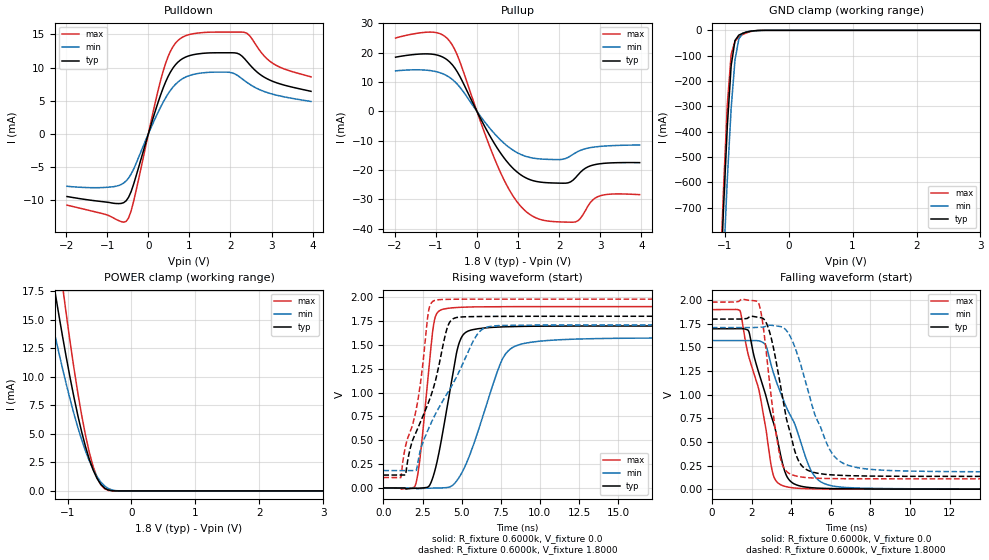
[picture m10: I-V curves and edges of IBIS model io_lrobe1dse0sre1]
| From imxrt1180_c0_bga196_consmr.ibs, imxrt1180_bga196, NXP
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[Model]  io_lrobe1dse0sre1
|   Model io_lrobe1dse0sre1
| This model was characterised for following simulation conditions:
| External (pad) voltage:
|   - Typ: 1.8V,   - Min: 1.71V,   - Max: 1.98V
| Library cells for typ/min/max conditions are connected as defined below:
|  PAD_IO - External Pad
|  ipp_do - Core Input
|  ipp_obe - Output Buffer Enable
|  ASRCN3V3[3] - NC
|  ASRCN3V3[4] - NC
|  ASRCP3V3[4] - NC
|  REFAPBIAS3V3 - gnde
|  REFBAMPL3V3 - vdd1v8
|  REFCAMPH3V3 - vdd1v8
|  REFDNBIAS3V3 - vdd1v8
|  REFH3V3 - REFH3V3
|  REFL3V3 - REFL3V3
|  gnde - gnde
|  ipp_dse - gnde
|  ipp_ina235_3v - NC
|  ipp_ina40_3v - NC
|  ipp_ina_mux - NC
|  ipp_ind - NC
|  ipp_ind_1p8v - NC
|  ipp_ind_3v - NC
|  ipp_sre - vdd
|  vdd - vdd
|  vdd1v8 - vdd1v8
|  vdda - vdde3v3
|  vdde3v3 - vdde3v3
| All other pins connected to ground
Model_type I/O
Polarity   Non-Inverting
Enable   Active-High
Vinl =   0.5400V
Vinh =   1.2600V
Vmeas =  0.9000V
Cref =   15.0000pF
Rref =   0.6000k
Vref =   0.0V
C_comp   3.9800pF   3.7960pF   4.1051pF
|C_comp_pullup   0.3206pF   0.4279pF   0.2788pF
|C_comp_pulldown   2.2503pF   2.3237pF   2.0515pF
[Model Spec]
| variable   typ   min   max
Vinh   1.2600V   NA   NA
Vinl   0.5400V   NA   NA
Vref   0.0V   0.0V   0.0V
Cref   15.0000pF   15.0000pF   15.0000pF
Rref   0.6000k   0.6000k   0.6000k
[Receiver Thresholds]
Vcross_high  =   0.0V
Vcross_low  =   0.0V
Vdiff_ac  =   0.0V
Vdiff_dc  =   0.0V
Tdiffslew_ac  =   0.0S
[Temperature Range]   25.0000   0.1250k   -40.0000
[Voltage Range]   1.8000V   1.7100V   1.9800V
[Pullup Reference]   1.8000V   1.7100V   1.9800V
[Pulldown Reference]   0.0V   0.0V   0.0V
[POWER Clamp Reference]   1.8000V   1.7100V   1.9800V
[GND Clamp Reference]   0.0V   0.0V   0.0V
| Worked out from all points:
|   slope of the pulldown table from 0 to 0.27 V, typ, clamps not added: 50.4 ohm
|   slope of the pullup table from 0 to 0.27 V, typ, clamps not added: 37.3 ohm
|   GND clamp passes 1 mA (typ) near -0.50 V on its own axis
|   POWER clamp passes 1 mA (typ) near -0.53 V on its own axis
|   rising waveform, R_fixture 0.6000k, V_fixture 0.0: 20-80 % time 1.09ns typ, 1.92ns min, 679ps max; typ from 0 V to 1.7 V
|   rising waveform, R_fixture 0.6000k, V_fixture 1.8000: 20-80 % time 1.97ns typ, 2.8ns min, 1.22ns max; typ from 0.135 V to 1.8 V
|   falling waveform, R_fixture 0.6000k, V_fixture 0.0: 20-80 % time 1.3ns typ, 1.7ns min, 1.16ns max; typ from 1.7 V to 0 V
|   falling waveform, R_fixture 0.6000k, V_fixture 1.8000: 20-80 % time 966ps typ, 1.43ns min, 661ps max; typ from 1.8 V to 0.135 V
[Pulldown]
|Voltage   I(typ)   I(min)   I(max)
-1.98V    -9.436mA   -7.895mA   -10.73mA
-840mV    -10.46mA   -7.944mA   -12.69mA
-600mV    -10.36mA   -7.401mA   -13.31mA
-480mV    -9.541mA   -6.639mA   -12.66mA
-360mV    -7.618mA   -5.325mA   -10.21mA
360mV     6.913mA    4.777mA    9.449mA
600mV     9.944mA    7.064mA    13.16mA
840mV     11.38mA    8.356mA    14.62mA
1.92V     12.24mA    9.319mA    15.36mA
2.34V     11.36mA    8.042mA    15.32mA
3V        8.003mA    6.042mA    10.77mA
3.96V     6.425mA    4.891mA    8.61mA
[Pullup]
|Voltage   I(typ)   I(min)   I(max)
-1.98V    18.49mA    13.82mA    25.02mA
-1.08V    19.49mA    13.79mA    27.02mA
-660mV    16.8mA     11.52mA    23.88mA
-420mV    12.05mA    8.333mA    17.13mA
180mV     -4.921mA   -3.425mA   -7.113mA
600mV     -14.73mA   -10.11mA   -21.67mA
960mV     -20.51mA   -13.95mA   -30.55mA
1.32V     -23.46mA   -15.83mA   -35.49mA
2.04V     -24.51mA   -16.44mA   -37.74mA
2.4V      -22.64mA   -14.15mA   -37.73mA
2.94V     -18mA      -12.04mA   -29.13mA
3.96V     -17.5mA    -11.48mA   -28.43mA
[GND_clamp]
|Voltage   I(typ)   I(min)   I(max)
-1.98V    -7.543A    -7.6A      -7.897A
-1.08V    -1.077A    -1.286A    -1.025A
-1.02V    -705.3mA   -921.3mA   -628.8mA
-960mV    -377.1mA   -587.4mA   -291.7mA
-900mV    -139.2mA   -307mA     -94.38mA
-840mV    -40.12mA   -117mA     -42.82mA
-780mV    -18.81mA   -33.95mA   -26.13mA
-720mV    -11.86mA   -11.44mA   -16.78mA
-660mV    -7.061mA   -5.737mA   -9.992mA
-540mV    -1.684mA   -1.901mA   -2.15mA
-420mV    -207.1uA   -403.7uA   -160.6uA
3.96V     0A         0A         0A
[POWER_clamp]
|Voltage   I(typ)   I(min)   I(max)
-1.98V    46.79mA    35.95mA    61.44mA
-1.32V    21.78mA    16.85mA    28.96mA
-1.2V     17.57mA    13.71mA    23.37mA
-1.08V    13.59mA    10.75mA    18.03mA
-1.02V    11.71mA    9.354mA    15.49mA
-900mV    8.21mA     6.76mA     10.75mA
-720mV    3.899mA    3.511mA    4.896mA
-600mV    1.839mA    1.889mA    2.143mA
-540mV    1.103mA    1.267mA    1.197mA
-420mV    244.5uA    429.3uA    190.7uA
-180mV    281nA      5.272uA    27.6nA
3.96V     0A         0A         0A
[Ramp]
| variable   typ   min   max
dV/dt_r  1.0188/1.0912n   0.9441/1.9229n   1.1406/0.6795n
dV/dt_f  0.9990/0.9660n   0.9166/1.4322n   1.1224/0.6606n
R_load = 0.6000k
[Rising Waveform]
R_fixture= 0.6000k
V_fixture= 0.0
V_fixture_min= 0.0
V_fixture_max= 0.0
|time   V(typ)   V(min)   V(max)
0s        119.2nV    3.183uV    128.2nV
2.063ns   -3.039mV   -887.6uV   37.74mV
2.356ns   -1.387mV   -6.165mV   333.8mV
3.214ns   137.3mV    -1.33mV    1.716V
3.927ns   709.8mV    2.224mV    1.878V
4.705ns   1.44V      78.98mV    1.892V
5.116ns   1.609V     191.9mV    1.895V
7.59ns    1.688V     1.346V     1.9V
9.222ns   1.694V     1.522V     1.901V
60ns      1.698V     1.573V     1.901V
[Rising Waveform]
R_fixture= 0.6000k
V_fixture= 1.8000
V_fixture_min= 1.7100
V_fixture_max= 1.9800
|time   V(typ)   V(min)   V(max)
0s        135mV      182.4mV    109.3mV
1.117ns   134.1mV    182.3mV    109.1mV
1.414ns   135.9mV    181.8mV    437.2mV
2.236ns   640.5mV    302.7mV    950.7mV
2.895ns   901.5mV    624.7mV    1.861V
3.384ns   1.163V     792.7mV    1.97V
4.326ns   1.756V     1.059V     1.978V
5.954ns   1.797V     1.599V     1.979V
7.058ns   1.798V     1.698V     1.98V
60ns      1.8V       1.71V      1.98V
[Falling Waveform]
R_fixture= 0.6000k
V_fixture= 0.0
V_fixture_min= 0.0
V_fixture_max= 0.0
|time   V(typ)   V(min)   V(max)
0s        1.698V     1.573V     1.901V
1.408ns   1.699V     1.573V     1.891V
1.841ns   1.677V     1.573V     1.415V
2.381ns   1.22V      1.569V     1.04V
2.672ns   1.026V     1.536V     699.1mV
3.089ns   711.5mV    1.239V     152.7mV
3.902ns   96.71mV    802.5mV    19.44mV
5.191ns   12.86mV    134.2mV    3.036mV
6.781ns   3.764mV    17.44mV    508.1uV
60ns      7.748uV    15.44uV    4.597uV
[Falling Waveform]
R_fixture= 0.6000k
V_fixture= 1.8000
V_fixture_min= 1.7100
V_fixture_max= 1.9800
|time   V(typ)   V(min)   V(max)
0s        1.8V       1.71V      1.98V
2.333ns   1.819V     1.713V     1.977V
2.594ns   1.805V     1.716V     1.71V
2.863ns   1.696V     1.736V     1.212V
3.442ns   1.113V     1.722V     337.9mV
3.81ns    699.6mV    1.665V     179.2mV
4.485ns   260.4mV    1.313V     129.4mV
6.053ns   151mV      381.8mV    111.9mV
8.046ns   138.4mV    209mV      109.5mV
60ns      135mV      182.4mV    109.3mV
